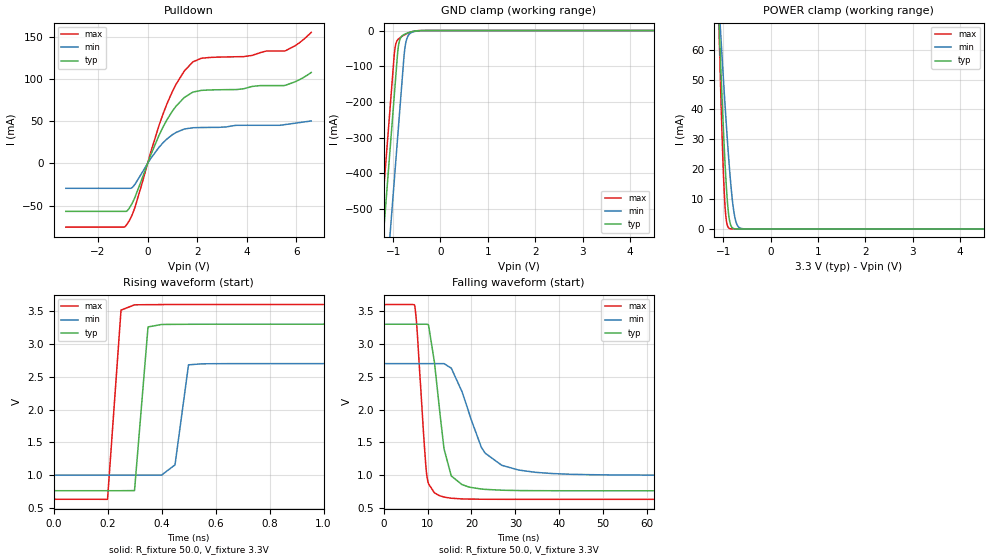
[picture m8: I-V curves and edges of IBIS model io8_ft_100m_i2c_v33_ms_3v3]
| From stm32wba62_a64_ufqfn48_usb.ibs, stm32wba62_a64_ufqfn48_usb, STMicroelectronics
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[Model]   io8_ft_100m_i2c_v33_ms_3v3
Model_type I/O_open_drain
Polarity   Non-Inverting
Enable   Active-Low
| CAP_THRESHOLD on pad IOFT is "UDTCAPC" :
| Rising=30.0% of vddiom   Falling=70.0% of vddiom
| C_comp min and max val. don't necessarily correlate with the min and max pvt
| but are the smallest and greatest pad capacitance found.
| var   typ   min   max
C_comp   3.81167pF  3.70520pF  3.86896pF
|C_comp_pulldown   3.81167pF  3.70520pF  3.86896pF
Vinl = 1.35V
Vinh = 1.8V
Vmeas = 1.65V   | Reference voltage for timing measurements
Cref  = 50.0pF   | Timing specification test load capacitance value
Rref  = 1.0MOhm   | Timing specification test load resistance value
Vref  = 1.815V   | Timing specification test load voltage
[Model Spec]
| TIME_THRESHOLD on pin ZII2CV11 is "CMOS" :
| Rising=50.0% of vdd   Falling=50.0% of vdd
Vinl 1.28450V 1.07450V 1.37050V
Vinh 1.79550V 1.51850V 1.89950V
| variable   typ   min   max
[Temperature Range] 25.0 140.0 -40.0
| variable   typ   min   max
[Voltage Range] 3.3V 2.7V 3.6V
| variable   typ   min   max
[POWER Clamp Reference] 3.3V 2.7V 3.6V
| variable   typ   min   max
[GND Clamp Reference] 0V 0V 0V
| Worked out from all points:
|   slope of the pulldown table from 0 to 0.495 V, typ, clamps not added: 14 ohm
|   GND clamp passes 1 mA (typ) near -0.51 V on its own axis
|   POWER clamp passes 1 mA (typ) near -0.83 V on its own axis
|   rising waveform, R_fixture 50.0, V_fixture 3.3V: 20-80 % time 30.5ps typ, 33.4ps min, 30.9ps max; typ from 0.764 V to 3.3 V
|   falling waveform, R_fixture 50.0, V_fixture 3.3V: 20-80 % time 2.88ns typ, 5.81ns min, 1.7ns max; typ from 3.3 V to 0.764 V
[POWER Clamp]
-3.3V     1.123A     753mA      1.645A
-1.09V    69.42mA    75.17mA    67.14mA
-1.08V    65.31mA    72.42mA    61.23mA
-1.06V    57.23mA    66.98mA    49.77mA
-1.01V    38.06mA    53.68mA    24.29mA
-970mV    24.36mA    43.46mA    9.575mA
-930mV    13.06mA    33.74mA    2.352mA
-870mV    3.065mA    20.56mA    165.9uA
-810mV    418.4uA    10.06mA    10.3uA
-760mV    69.41uA    4.321mA    1.009uA
-630mV    611.5nA    197uA      2.727nA
6.6V      0A         0A         0A
[GND Clamp]
-3.3V     -4.134A    -4.372A    -4.018A
-1.59V    -1.227A    -1.465A    -1.111A
-1.25V    -648.9mA   -886.9mA   -533mA
-980mV    -189.9mA   -427.9mA   -74mA
-960mV    -155.9mA   -393.9mA   -48.8mA
-910mV    -70.86mA   -308.9mA   -27.2mA
-880mV    -37.23mA   -257.9mA   -22.76mA
-770mV    -11.28mA   -71.59mA   -12.95mA
-730mV    -8.709mA   -32.74mA   -10.07mA
-630mV    -4.122mA   -6.943mA   -4.354mA
-370mV    -42.68uA   -212.2uA   -13.03uA
6.6V      2.311nA    506.4nA    1.057nA
| variable   typ   min   max
[Pullup Reference] 3.3V 2.7V 3.6V
| variable   typ   min   max
[Pulldown Reference] 0V 0V 0V
[Pulldown]
-3.3V     -56.7mA    -29.42mA   -75.36mA
-860mV    -56.67mA   -29.42mA   -72.94mA
-520mV    -40.69mA   -25.01mA   -52.64mA
460mV     33.25mA    19.09mA    44.92mA
800mV     52.54mA    29.36mA    71.75mA
1.14V     67.41mA    36.49mA    93.2mA
1.48V     77.97mA    40.67mA    109.3mA
1.83V     84.38mA    42.18mA    120.1mA
2.17V     86.37mA    42.45mA    124.3mA
3.88V     88.31mA    45.1mA     126.3mA
5.54V     92.28mA    45.89mA    133mA
6.6V      107.5mA    50.2mA     155mA
[Ramp]
dV/dt_r 1.52155V/251.33128ps 1.01896V/341.1356ps 1.7797V/235.87043ps
dV/dt_f 1.52157V/2.58047ns 1.019V/5.68168ns 1.77971V/1.69563ns
R_load = 50.0
| Removed startup time: 0s 0s 0s  .
| Removed end time: 1.65ns.
[Rising Waveform]
R_fixture   = 50.0
V_fixture   = 3.3V
V_fixture_min = 2.7V
V_fixture_max = 3.6V
0s        764mV      1.002V     633.8mV
200ps     764mV      1.002V     632.9mV
250ps     764mV      1.002V     3.514V
300ps     766.2mV    1.002V     3.595V
350ps     3.258V     1.002V     3.597V
400ps     3.296V     1.001V     3.599V
450ps     3.298V     1.158V     3.6V
500ps     3.299V     2.681V     3.6V
600ps     3.3V       2.698V     3.6V
1.65ns    3.3V       2.7V       3.6V
| Removed startup time: 0s 0s 0s  .
| Removed end time: 188.4ns.
[Falling Waveform]
R_fixture   = 50.0
V_fixture   = 3.3V
V_fixture_min = 2.7V
V_fixture_max = 3.6V
0s        3.3V       2.7V       3.6V
7.05ns    3.3V       2.7V       3.588V
7.6ns     3.3V       2.7V       3.227V
9.9ns     3.299V     2.7V       965.3mV
11.55ns   2.728V     2.7V       735mV
13.75ns   1.404V     2.7V       668.3mV
15.4ns    990.2mV    2.631V     650.6mV
23.1ns    785.6mV    1.338V     635mV
30.75ns   767.6mV    1.08V      633.9mV
188.4ns   764mV      1.002V     633.8mV
